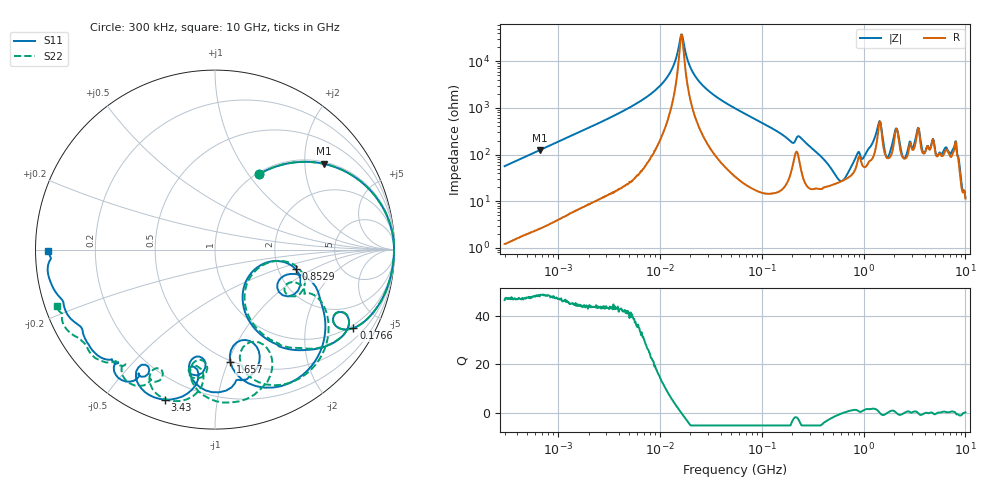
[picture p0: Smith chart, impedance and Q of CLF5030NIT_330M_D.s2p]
! S-Parameter Data Generated by TDK Corporation
! Copyright(C) 2019 TDK Corporation.
! All Rights Reserved.
! TDK P/N: CLF5030NIT-330M-D (Inductor)
! Property: L=33uH at 100kHz
! Size(LxWxT): 5.3x5x2.7mm
! Model Type: s2p (Touchstone File Format Version 1.0)
! Frequency: DC=Yes Start=0.3MHz Stop=10000MHz 802points Log-sweep
! Model Generated on May 10, 2019
! Port Assignments:
!  1 ---@@@--- 2
! Applicable Conditions:
!  Temperature = 25 degC
!  DC Bias Current = 0 A
!  Small Signal Operation
! Terms and conditions regarding TDK Simulation Models
! (1)This simulation model is being provided solely for informational purposes. Please refer to the specifications of the products in terms of detailed characteristics of such products.
! (2)In no event shall TDK Corporation of any of its subsidiaries be liable for any loss or damage arising, directly or indirectly,
!  From any information contained in this simulation model, including, but not limited to loss or damages arising from any inaccuracies, omissions or errors in connection with such information.
! (3)Any and all copyrights on this simulation model are owned by TDK Corporation.
!  Duplication or redistribution of this simulation model without prior written permission from TDK Corporation is prohibited.
! (4)This simulation model is subject to any modification or change without any prior notice.
! (5)Neither TDK Corporation nor any of its subsidiaries shall make any warranty, express or implied,
!  Including but not limited to the correctness, implied warranties of merchantability and fitness for a particular purpose with respect to this simulation models.
! (6)The use of this simulation model shall be deemed to have consented to the terms and conditions hereof.
# Hz S MA R 50
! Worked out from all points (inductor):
!   801 points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, 300 kHz to 10 GHz, reference 50 ohm
!   read as one part in series: L = 29.9 uH near 318.3 kHz
!   highest Q = 48.4 at 663.1 kHz (marker M1), where L = 29.8 uH
!   self-resonance near 16.27 MHz
!   S11 on the Smith chart (normalised r, x): 300 kHz: 1.02, +1.13; 176.6 MHz: 0.88, -3.59; 852.9 MHz: 2.50, -0.70; 1.657 GHz: 0.49, -1.02; 3.43 GHz: 0.10, -0.72; 10 GHz: 0.04, -0.01
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300000  0.488 59.6  0.8625 -29.1  0.8623 -29.1  0.4878 59.6
663069  0.7712 38.3  0.6207 -50.5  0.6208 -50.5  0.7712 38.3
1713600  0.9481 17.2  0.2969 -71.5  0.2969 -71.5  0.9481 17.2
9671944  0.997 1.7  0.03647 -84.7  0.03649 -84.8  0.9971 1.7
1.649435e7  0.9974 -0.7  0.002669 9.8  0.002683 9.9  0.9974 -0.7
2.378472e7  0.9968 -2.4  0.02535 81.3  0.02534 81.3  0.9969 -2.4
5.477226e7  0.9913 -8.1  0.1009 80.0  0.1009 80.0  0.9914 -8.1
1.765741e8  0.8866 -29.5  0.3795 54.5  0.3795 54.5  0.8865 -29.5
3.126428e8  0.787 -44.7  0.529 38.2  0.529 38.2  0.7829 -44.7
5.663179e8  0.341 -62.7  0.7585 -6.8  0.7584 -6.8  0.3449 -61.0
6.904357e8  0.2407 -32.5  0.7491 -27.1  0.7491 -27.1  0.2505 -31.2
8.528959e8  0.4638 -13.7  0.5814 -52.4  0.5814 -52.4  0.4772 -12.5
1.180962e9  0.6652 -26.9  0.4396 -77.5  0.4393 -77.5  0.6048 -24.6
1.43752e9  0.8537 -57.6  0.1287 -66.0  0.1286 -66.0  0.8591 -53.9
1.657186e9  0.6306 -82.2  0.3924 -41.9  0.3921 -41.9  0.6468 -77.3
1.767019e9  0.5261 -74.0  0.4354 -67.3  0.4349 -67.3  0.5518 -69.1
2.08171e9  0.7363 -80.1  0.1334 -82.7  0.1328 -82.3  0.8507 -78.0
2.568366e9  0.6127 -101.0  0.341 -81.5  0.3409 -81.4  0.6226 -98.7
3.429941e9  0.8816 -108.5  0.08494 -102.8  0.08525 -102.5  0.8729 -104.6
5.607117e9  0.845 -131.7  0.1411 -124.2  0.1418 -124.0  0.8358 -129.6
8.211115e9  0.896 -161.7  0.02512 -105.7  0.02491 -107.6  0.9316 -156.3
1e10  0.9287 -179.4  0.05128 -92.7  0.05115 -92.6  0.9345 -160.4
